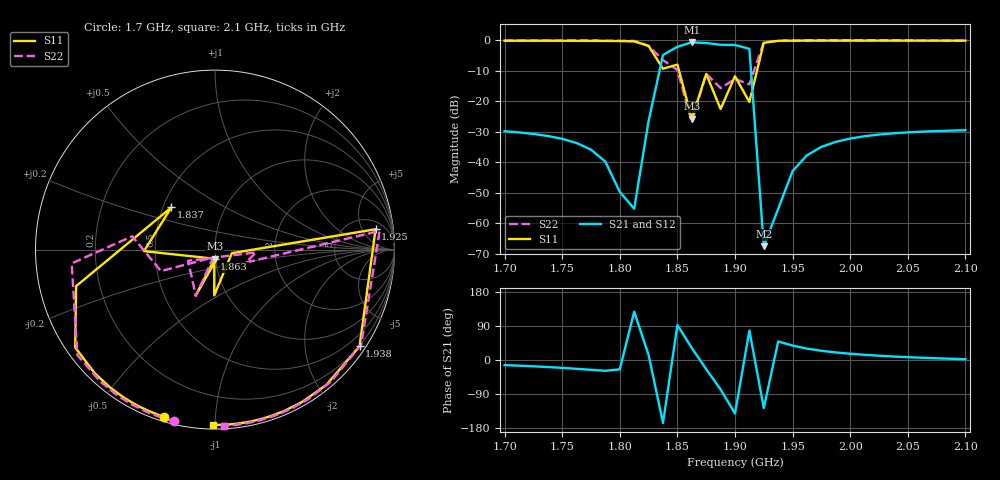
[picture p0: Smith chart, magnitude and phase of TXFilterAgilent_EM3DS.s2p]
!AWR Design Environment (2469) Mon Oct 04 19:05:12 2004
!freq-unit  param-type  data-format  keyword  impedance-ohms
# GHz  S  MA  R  50
!Freq  MagS11  AngS11  MagS21  AngS21  MagS12  AngS12  MagS22  AngS22
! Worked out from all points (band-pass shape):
!   33 points, 1.7 GHz to 2.1 GHz, reference 50 ohm
!   highest |S21| = -0.75 dB at 1.863 GHz (marker M1); lowest = -67.6 dB at 1.925 GHz (marker M2)
!   |S21| within 3 dB of the highest: 1.843 GHz to 1.913 GHz (69.78 MHz wide, 3.72 % of centre)
!   lowest |S11| = -25.8 dB at 1.863 GHz (marker M3), VSWR 1.11, Z = 49.6 - j5.08 ohm
!   |S11| at or under -10 dB: 1.851 GHz to 1.919 GHz (67.78 MHz wide, 3.6 % of centre)
!   |S22| runs from -27.0 to -0.1 dB; largest |S21 - S12| = 0
!   S11 on the Smith chart (normalised r, x): 1.7 GHz: 0.02, -0.74; 1.837 GHz: 0.55, +0.29; 1.863 GHz: 0.99, -0.10; 1.925 GHz: 8, +9; 1.938 GHz: 0.19, -3.28; 2.1 GHz: 0.02, -0.99
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1.7  0.9739 -106.9  0.03195 -13.4  0.03195 -13.4  0.9827 -103.4
1.75  0.971 -115.3  0.02401 -20.8  0.02401 -20.8  0.9809 -111.8
1.775  0.968 -122.2  0.01596 -26.0  0.01596 -26.0  0.9791 -118.8
1.7875  0.9654 -127.2  0.01012 -28.5  0.01012 -28.5  0.9773 -123.8
1.8  0.9609 -134.1  0.003245 -24.7  0.003245 -24.7  0.9741 -130.9
1.8125  0.951 -145.0  0.001714 127.4  0.001714 127.4  0.9659 -142.5
1.825  0.8001 -165.3  0.04715 13.2  0.04715 13.2  0.8022 -174.5
1.8375  0.3382 135.9  0.5684 -166.1  0.5684 -166.1  0.4673 170.9
1.85  0.3957 -178.8  0.7738 92.1  0.7738 92.1  0.3239 -158.3
1.8625  0.05109 -91.8  0.917 31.6  0.917 31.6  0.0448 -102.9
1.875  0.2783 -112.8  0.893 -24.2  0.893 -24.2  0.2792 -112.5
1.8875  0.07403 -93.1  0.8354 -77.6  0.8354 -77.6  0.1626 -157.4
1.9  0.2552 -91.0  0.8291 -141.3  0.8291 -141.3  0.2297 -3.8
1.9125  0.09614 -11.9  0.7159 77.7  0.7159 77.7  0.1873 -22.5
1.925  0.9019 7.2  0.0004178 -126.9  0.0004178 -126.9  0.9231 6.5
1.9375  0.9691 -33.8  0.001708 48.9  0.001708 48.9  0.9713 -33.0
1.95  0.976 -50.5  0.00711 38.0  0.00711 38.0  0.9789 -48.7
1.9625  0.9779 -60.2  0.01291 30.1  0.01291 30.1  0.9815 -57.9
1.975  0.9784 -66.8  0.0177 24.3  0.0177 24.3  0.9826 -64.1
2  0.9783 -75.4  0.02428 16.5  0.02428 16.5  0.9833 -72.4
2.0375  0.9775 -83.1  0.02955 9.3  0.02955 9.3  0.9834 -79.8
2.1  0.9763 -90.6  0.03317 2.1  0.03317 2.1  0.983 -87.1
